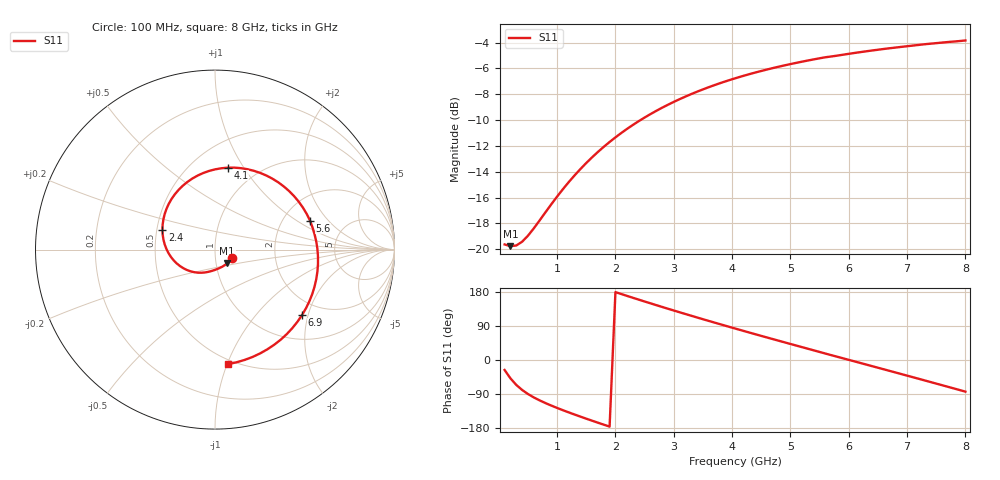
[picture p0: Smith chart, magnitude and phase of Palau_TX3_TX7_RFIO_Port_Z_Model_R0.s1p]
! Created Wed Jul 15 11:54:48 2020
! Palau TX3/TX7 RFIO Port Impedance Model.
! Revision		: R0.
! Impedance Mode 	: Balanced Differential-Mode.
! Impedance Format 	: Series Equivalent Differential Impedance (SEDZ).
# hz S ma R 100
! 1 Port Network Data from SP1.SP block
! freq  magS11  angS11
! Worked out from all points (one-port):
!   80 points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, 100 MHz to 8 GHz, reference 100 ohm
!   lowest |S11| = -19.8 dB at 200 MHz (marker M1), VSWR 1.23, Z = 113 - j17.6 ohm
!   |S11| at or under -10 dB: start of sweep to 2.43 GHz
!   S11 on the Smith chart (normalised r, x): 100 MHz: 1.20, -0.11; 2.4 GHz: 0.54, +0.13; 4.1 GHz: 0.74, +0.85; 5.6 GHz: 2.80, +1.31; 6.9 GHz: 1.58, -1.83; 8 GHz: 0.46, -1.01
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1e8  0.1044 -26.3
2e8  0.1028 -48.5
3e8  0.1034 -65.7
5e8  0.1128 -89.7
8e8  0.139 -113.6
1.1e9  0.1708 -132.5
1.3e9  0.1932 -143.9
1.6e9  0.2269 -160.2
2.1e9  0.2817 174.1
2.4e9  0.3132 159.3
2.7e9  0.3432 144.8
3.1e9  0.3808 126.0
3.6e9  0.4238 103.2
3.9e9  0.4473 89.8
4.1e9  0.4621 81.0
4.3e9  0.4762 72.3
4.6e9  0.4962 59.4
4.8e9  0.5087 50.8
5.1e9  0.5264 38.1
5.6e9  0.5533 17.0
5.9e9  0.5659 4.6
6.1e9  0.575 -3.7
6.5e9  0.5917 -20.3
6.9e9  0.6068 -37.0
7.1e9  0.614 -45.4
7.4e9  0.6244 -58.1
7.6e9  0.6306 -66.5
8e9  0.6427 -83.5
